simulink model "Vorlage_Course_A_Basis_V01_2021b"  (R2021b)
settings: Solver=FixedStepAuto  StartTime=0.0  StopTime=inf  FixedStep=1e-3  RelTol=1e-3
undefined symbols (not defined in the file): bin2dec
libraries: simulink x9, instrumentseriallib x3, eeGeneralControl x1

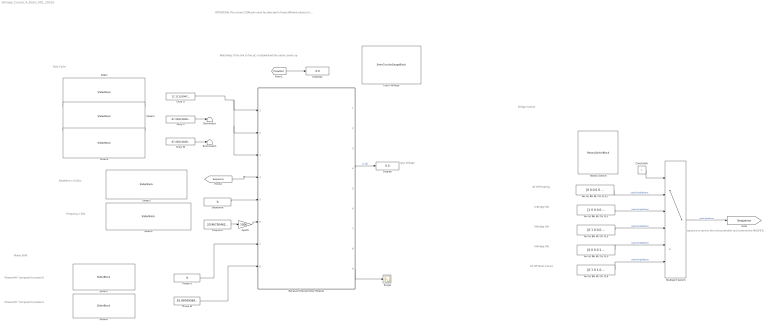
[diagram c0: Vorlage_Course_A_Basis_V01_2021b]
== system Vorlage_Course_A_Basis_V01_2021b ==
  note: Sequence is sent to the microcontroller and controls the MOSFETs
  note: Duty Cycle
  note: Phase Shift
  note: All Off Floating
  note: Watchdog: If the link to the µC is established the value counts up
  note: ATTENTION: The correct COM port must be selected in three different places in the receiver and transmitter module. (Available interfaces, see Windows Control Panel)
  note: Deadtime x 6,25ns
  note: Frequency / kHz
  note: Phaseshift °compared to phase U
  note: Phaseshift °compared to phase U
  note: U-Bridge ON
  note: V-Bridge ON
  note: V-Bridge ON
  note: All Off Short Circuit
  note: Bridge Control
  note: Input Voltage
  AH AL BH BL CH CL1 : Constant  Value=[1 0 0 0 0 0]  SampleTime=-1
  AH AL BH BL CH CL11 : Constant  Value=[0 0 0 0 0 0]  SampleTime=-1
  AH AL BH BL CH CL2 : Constant  Value=[0 1 0 0 0 0]  SampleTime=-1
  AH AL BH BL CH CL3 : Constant  Value=[0 0 0 0 1 0]  SampleTime=-1
  AH AL BH BL CH CL4 : Constant  Value=[0 1 0 1 0 1]
  Constant6 : Constant  OutDataTypeStr=uint8
  Deadtime : Constant  Value=0  OutDataTypeStr=uint16
  Display : Display
  Display1 : Display
  Duty U : Constant  Value=11.11110947376479
  Duty V : Constant  Value=67.2652182831598
  Duty W : Constant  Value=67.2652182831598
  Frequenz : Constant  Value=20.96730462519936  OutDataTypeStr=uint16
  Gain6 : Gain  Gain=1000
  Input Voltage : SemiCircularGaugeBlock  ScaleMax=25
  Multiport Switch : MultiPortSwitch  Inputs=5  DiagnosticForDefault=None
  Phase V : Constant  Value=0  OutDataTypeStr=uint16
  Phase W : Constant  Value=55.99769364620121  OutDataTypeStr=uint16
  Receiver/Transimmter Module : Subsystem
  Rotary Switch : RotarySwitchBlock
  Scope : Scope
  Slider : SliderBlock  TickInterval=20
  Slider1 : SliderBlock  TickInterval=20
  Slider2 : SliderBlock  TickInterval=20
  Slider3 : SliderBlock  ScaleMax=500  TickInterval=50
  Slider4 : SliderBlock  ScaleMin=1  ScaleMax=50  TickInterval=10
  Slider5 : SliderBlock  ScaleMax=180  TickInterval=20
  Slider6 : SliderBlock  ScaleMax=180  TickInterval=20
  Terminator : Terminator
  Terminator1 : Terminator
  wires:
  AH AL BH BL CH CL1/1 -> Multiport Switch/3  "switchingPattern"
  AH AL BH BL CH CL11/1 -> Multiport Switch/2  "switchingPattern"
  AH AL BH BL CH CL2/1 -> Multiport Switch/4  "switchingPattern"
  Multiport Switch/1 -> [Sequence]  "switchpattern"
  AH AL BH BL CH CL3/1 -> Multiport Switch/5  "switchingPattern"
  Constant6/1 -> Multiport Switch/1
  AH AL BH BL CH CL4/1 -> Multiport Switch/6  "switchingPattern"
  [Sequence] -> Receiver/Transimmter Module/4(Sequence UH UL VH VL WH WL)
  [Counter] -> Display1/1
  Duty U/1 -> Receiver/Transimmter Module/2(Duty V [%]), Receiver/Transimmter Module/3(Duty W [%]), Receiver/Transimmter Module/1(Duty U [%])
  Deadtime/1 -> Receiver/Transimmter Module/5(Deadtime [x6,25n])
  Frequenz/1 -> Gain6/1
  Gain6/1 -> Receiver/Transimmter Module/6(Frequency [Hz])
  Phase V/1 -> Receiver/Transimmter Module/7(Phase V - U [°])
  Phase W/1 -> Receiver/Transimmter Module/8(Phase W - U [°])
  Duty V/1 -> Terminator/1
  Duty W/1 -> Terminator1/1
  Receiver/Transimmter Module/4(U_ZK [V]) -> Display/1  "U_ZK"
  Receiver/Transimmter Module/9(Analog Sig) -> Scope/1

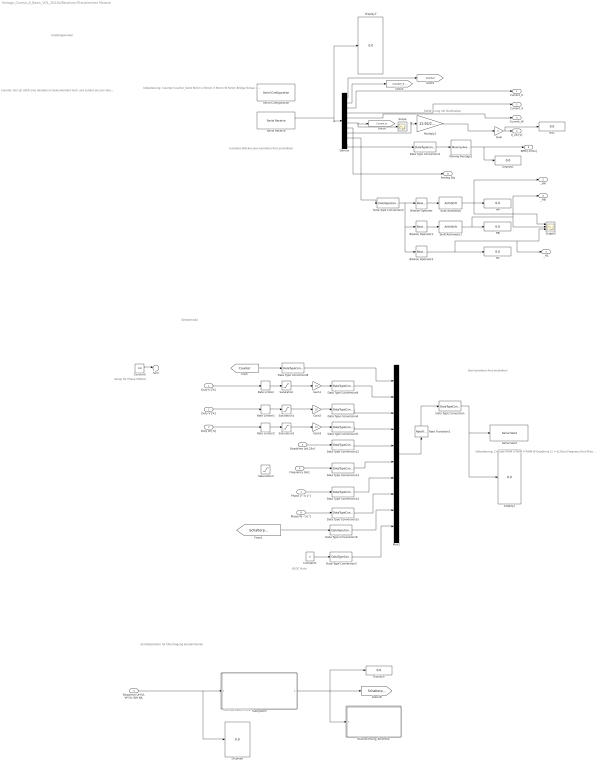
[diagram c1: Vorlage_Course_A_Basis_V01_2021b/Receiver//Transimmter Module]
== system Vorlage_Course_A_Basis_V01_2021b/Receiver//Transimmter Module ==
  note: BLDC Auto
  note: Setup für Phase-Shifted
  note: Counter: Der µC zählt eine Variable im Sekundentakt hoch und sendet sie zum Host Counter_Send: Der empfangene Wert wird wieder nach unten gesendet und sofort wieder empfangen Die Variable läuft ein mal im Kreis. Zählen beide Werte hoch ist alles in Ordnung. Zählt nur der Counter hoch bedeutet das, dass der Ursprungscounter nicht zurückgesendet wurde bzw. allgemein kein Daten von Simulink zum µC übertragen werden.
  note: Dekodierung: Counter Counter_Send Strom U Strom V Strom W Strom Bridge Torque U Zwischenkreis Hall Drehzahl
  note: Kalibrierung mit Oszilloskop
  note: Dekodierung: Counter PWM U PWM V PWM W Deadtime [1 = 6,25ns] Frequenz [Hz] Phase V PHase W Schaltsequenz BLDC Automatic
  note: Den korrekten Port einstellen!
  note: Sendemodul
  note: Empfangsmodul
  note: In beiden Blöcken den korrekten Port einstelllen!
  note: Schalterpattern für Übertragung komplrimieren
  note: Gibt das Pattern aus
  Duty U [%] : Inport
  Duty V [%] : Inport  Port=2
  Duty W [%] : Inport  Port=3
  Sequence UH UL VH VL WH WL : Inport  Port=4
  Deadtime [x6,25n] : Inport  Port=5
  Frequency [Hz] : Inport  Port=6
  Phase V - U [°] : Inport  Port=7
  Phase W - U [°] : Inport  Port=8
  Bitwise Operator : simulink/Logic and Bit Operations/Bitwise Operator  logicop=AND  UseBitMask=on  BitMask=bin2dec('00000100')  BitMaskRealWorld=Stored Integer
  Bitwise Operator1 : simulink/Logic and Bit Operations/Bitwise Operator  logicop=AND  UseBitMask=on  BitMask=bin2dec('00000010')  BitMaskRealWorld=Stored Integer
  Bitwise Operator2 : simulink/Logic and Bit Operations/Bitwise Operator  logicop=AND  UseBitMask=on  BitMask=bin2dec('00000001')  BitMaskRealWorld=Stored Integer
  Constant : Constant  Value=100
  Constant1 : Constant  Value=0
  Data Type Conversion{,3..5,8..9,12..16} (11 alike) : DataTypeConversion  OutDataTypeStr=uint16
  Data Type Conversion1 : DataTypeConversion  OutDataTypeStr=double
  Data Type Conversion2 : DataTypeConversion  OutDataTypeStr=uint8
  Demux : Demux  Outputs=10
  Display{1..2,5..7} (5 alike) : Display
  Gain : Gain
  Gain1 : Gain  Gain=10
  Gain2 : Gain  Gain=10
  Gain3 : Gain  Gain=10
  HA : Display
  HA1 : Display
  HB : Display
  HC : Display
  Moving Average1 : eeGeneralControl/Moving Average  VariantControl=Variant1  LabelModeActiveChoice=Discrete  f=2  x0=0  BufferSize=8192  Ts=-1
  Multiply1 : Gain  Gain=22.92/2366
  Mux2 : Mux  Inputs=10
  Rate Limiter : RateLimiter  RisingSlewLimit=200  FallingSlewLimit=-200
  Rate Limiter1 : RateLimiter  RisingSlewLimit=200  FallingSlewLimit=-200
  Rate Limiter2 : RateLimiter  RisingSlewLimit=200  FallingSlewLimit=-200
  Rate Transition1 : RateTransition  OutPortSampleTime=0.05
  Rückrechnung_Kontrolle : Subsystem
  Saturation : Saturate  UpperLimit=90  LowerLimit=0
  Saturation1 : Saturate  UpperLimit=90  LowerLimit=0
  Saturation2 : Saturate  UpperLimit=90  LowerLimit=0
  Saturation3 : Saturate  UpperLimit=100000  LowerLimit=1000
  Scope : Scope
  Scope3 : Scope  NumInputPorts=3
  Serial Configuration : instrumentseriallib/Serial Configuration  Priority=-200000  Port=COM22  ComPort=COM22  BaudRate=115000  DataBits=8  Parity=even  StopBits=1  ByteOrder=little-endian  FlowControl=none  Timeout=10  SimulateUsing=Interpreted execution  BlockInModel=on
  Serial Receive : instrumentseriallib/Serial Receive  Priority=1  Port=COM22  ComPort=COM22  DataType=uint16  SaveDataType=uint8  ToggleHeader=on  Header=['X']  ToggleTerminator=on  Terminator=Custom terminator  CustomTerminator=['Y']  ToggleDataSize=on  DataSize=[1 10]  EnableBlockingMode=off  ActionDataUnavailable=Output last received value  ActionWhenDataUnavailable=Output last received value  CustomValue=42  SampleTime=0.001  SimulateUsing=Interpreted execution  BlockInModel=on
  Serial Send : instrumentseriallib/Serial Send  Priority=1  Port=COM22  ComPort=COM22  Header=[]  Terminator=<none>  CustomTerminator=[]  EnableBlockingMode=off  SimulateUsing=Interpreted execution  BlockInModel=on
  Shift Arithmetic : ArithShift  BitShiftNumber=2  BitShiftDirection=Right
  Shift Arithmetic1 : ArithShift  BitShiftNumber=1  BitShiftDirection=Right
  Subsystem : Subsystem
  Sum : Sum  Inputs=|+-
  Current_U : Outport
  Current_V : Outport  Port=2
  Current_W : Outport  Port=3
  U_ZK [V] : Outport  Port=4
  _HA : Outport  Port=5
  _HB : Outport  Port=6
  _HC : Outport  Port=7
  " RPM [1/min]" : Outport  Port=8
  Analog Sig : Outport  Port=9
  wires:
  Demux/4 -> Current_V/1
  Data Type Conversion1/1 -> Moving Average1/1
  Serial Receive/1 -> Demux/1, Display7/1
  Demux/3 -> Current_U/1
  Moving Average1/1 -> " RPM [1/min]"/1, Display1/1
  Demux/5 -> Current_W/1
  Demux/6 -> Scope/1, [Current_In]
  Demux/2 -> [Counter_Send]
  Multiply1/1 -> Gain/1
  Demux/10 -> Data Type Conversion1/1
  Bitwise Operator1/1 -> Shift Arithmetic1/1
  Data Type Conversion2/1 -> Bitwise Operator2/1, Bitwise Operator1/1, Bitwise Operator/1
  Bitwise Operator/1 -> Shift Arithmetic/1
  Shift Arithmetic/1 -> _HA/1, Scope3/1, HA/1
  Shift Arithmetic1/1 -> _HB/1, Scope3/2, HB/1
  Bitwise Operator2/1 -> HC/1, _HC/1, Scope3/3
  Demux/8 -> Multiply1/1
  Demux/9 -> Data Type Conversion2/1
  Demux/1 -> [Counter]
  Data Type Conversion15/1 -> Mux2/8
  Data Type Conversion12/1 -> Mux2/5
  Data Type Conversion16/1 -> Mux2/9
  Data Type Conversion13/1 -> Mux2/6
  Data Type Conversion8/1 -> Mux2/1
  Data Type Conversion9/1 -> Mux2/2
  Rate Transition1/1 -> Data Type Conversion/1
  Mux2/1 -> Rate Transition1/1
  Gain1/1 -> Data Type Conversion9/1
  Duty U [%]/1 -> Rate Limiter/1
  Data Type Conversion/1 -> Display2/1, Serial Send/1
  Data Type Conversion14/1 -> Mux2/7
  Data Type Conversion3/1 -> Mux2/10
  [Counter] -> Data Type Conversion8/1
  Gain/1 -> HA1/1, U_ZK [V]/1
  Gain2/1 -> Data Type Conversion4/1
  Data Type Conversion4/1 -> Mux2/3
  Data Type Conversion5/1 -> Mux2/4
  Gain3/1 -> Data Type Conversion5/1
  Duty W [%]/1 -> Rate Limiter2/1
  Subsystem/1(Out1) -> Rückrechnung_Kontrolle/1(In1), [Schalterpattern], Display5/1
  Sequence UH UL VH VL WH WL/1 -> Display6/1, Subsystem/1(switchpattern)
  [Schalterpattern] -> Data Type Conversion16/1
  Rate Limiter/1 -> Saturation/1
  Rate Limiter1/1 -> Saturation1/1
  Rate Limiter2/1 -> Saturation2/1
  Constant/1 -> Sum/1
  Duty V [%]/1 -> Rate Limiter1/1
  Deadtime [x6,25n]/1 -> Data Type Conversion12/1
  Constant1/1 -> Data Type Conversion3/1
  Phase V - U [°]/1 -> Data Type Conversion14/1
  Phase W - U [°]/1 -> Data Type Conversion15/1
  Saturation/1 -> Gain1/1
  Saturation1/1 -> Gain2/1
  Saturation2/1 -> Gain3/1
  Frequency [Hz]/1 -> Data Type Conversion13/1
  Demux/7 -> Analog Sig/1

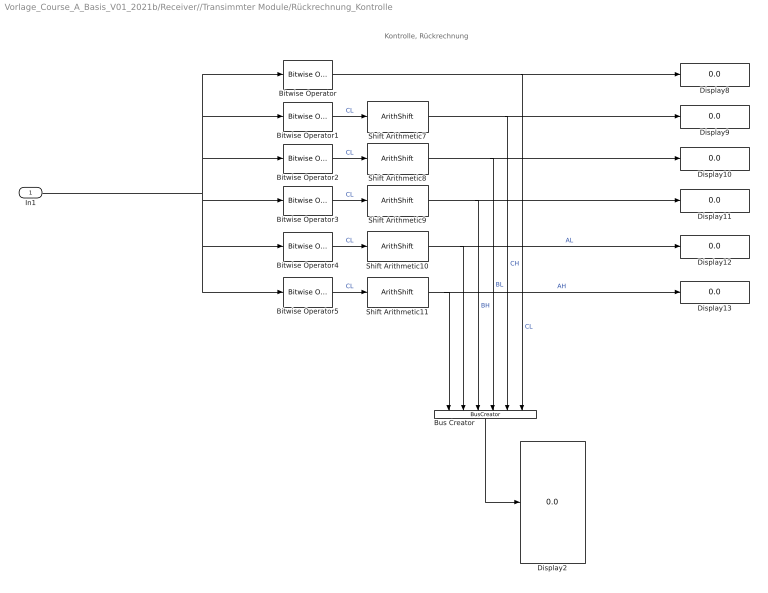
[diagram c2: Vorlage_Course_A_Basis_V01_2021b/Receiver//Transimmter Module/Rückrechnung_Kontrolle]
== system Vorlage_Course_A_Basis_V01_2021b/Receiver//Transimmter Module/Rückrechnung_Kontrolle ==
  note: Kontrolle, Rückrechnung
  In1 : Inport
  Bitwise Operator : simulink/Logic and Bit Operations/Bitwise Operator  logicop=AND  UseBitMask=on  BitMask=0x01  BitMaskRealWorld=Stored Integer
  Bitwise Operator1 : simulink/Logic and Bit Operations/Bitwise Operator  logicop=AND  UseBitMask=on  BitMask=0x02  BitMaskRealWorld=Stored Integer
  Bitwise Operator2 : simulink/Logic and Bit Operations/Bitwise Operator  logicop=AND  UseBitMask=on  BitMask=0x04  BitMaskRealWorld=Stored Integer
  Bitwise Operator3 : simulink/Logic and Bit Operations/Bitwise Operator  logicop=AND  UseBitMask=on  BitMask=0x08  BitMaskRealWorld=Stored Integer
  Bitwise Operator4 : simulink/Logic and Bit Operations/Bitwise Operator  logicop=AND  UseBitMask=on  BitMask=0x10  BitMaskRealWorld=Stored Integer
  Bitwise Operator5 : simulink/Logic and Bit Operations/Bitwise Operator  logicop=AND  UseBitMask=on  BitMask=0x20  BitMaskRealWorld=Stored Integer
  Bus Creator : BusCreator  Inputs=6
  Display{2,8..13} (7 alike) : Display
  Shift Arithmetic10 : ArithShift  BitShiftNumber=4  BitShiftDirection=Right
  Shift Arithmetic11 : ArithShift  BitShiftNumber=5  BitShiftDirection=Right
  Shift Arithmetic7 : ArithShift  BitShiftNumber=1  BitShiftDirection=Right
  Shift Arithmetic8 : ArithShift  BitShiftNumber=2  BitShiftDirection=Right
  Shift Arithmetic9 : ArithShift  BitShiftNumber=3  BitShiftDirection=Right
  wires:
  Shift Arithmetic8/1 -> Bus Creator/4, Display10/1  "BL"
  Shift Arithmetic9/1 -> Bus Creator/3, Display11/1  "BH"
  In1/1 -> Bitwise Operator/1, Bitwise Operator1/1, Bitwise Operator2/1, Bitwise Operator5/1, Bitwise Operator4/1, Bitwise Operator3/1
  Bitwise Operator2/1 -> Shift Arithmetic8/1  "CL"
  Shift Arithmetic7/1 -> Bus Creator/5, Display9/1  "CH"
  Shift Arithmetic10/1 -> Display12/1, Bus Creator/2  "AL"
  Bitwise Operator5/1 -> Shift Arithmetic11/1  "CL"
  Shift Arithmetic11/1 -> Display13/1, Bus Creator/1  "AH"
  Bitwise Operator/1 -> Bus Creator/6, Display8/1  "CL"
  Bus Creator/1 -> Display2/1
  Bitwise Operator1/1 -> Shift Arithmetic7/1  "CL"
  Bitwise Operator4/1 -> Shift Arithmetic10/1  "CL"
  Bitwise Operator3/1 -> Shift Arithmetic9/1  "CL"

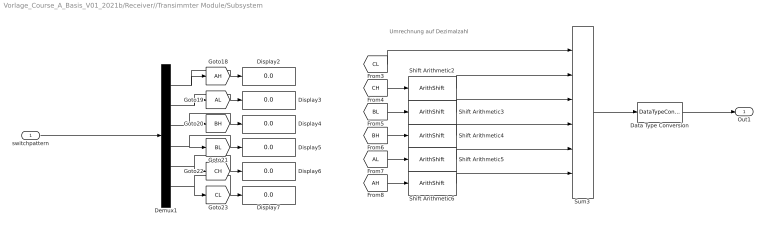
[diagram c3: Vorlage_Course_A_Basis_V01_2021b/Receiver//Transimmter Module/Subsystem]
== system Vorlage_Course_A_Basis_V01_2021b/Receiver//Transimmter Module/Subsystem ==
  note: Umrechnung auf Dezimalzahl
  switchpattern : Inport
  Data Type Conversion : DataTypeConversion  OutDataTypeStr=uint8
  Demux1 : Demux  Outputs=6
  Display{2..7} (6 alike) : Display
  Shift Arithmetic2 : ArithShift  BitShiftNumber=1  BitShiftDirection=Left
  Shift Arithmetic3 : ArithShift  BitShiftNumber=2  BitShiftDirection=Left
  Shift Arithmetic4 : ArithShift  BitShiftNumber=3  BitShiftDirection=Left
  Shift Arithmetic5 : ArithShift  BitShiftNumber=4  BitShiftDirection=Left
  Shift Arithmetic6 : ArithShift  BitShiftNumber=5  BitShiftDirection=Left
  Sum3 : Sum  Inputs=|++++++
  Out1 : Outport
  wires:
  [CL] -> Sum3/1
  Demux1/2 -> Display3/1, [AL]
  Demux1/4 -> [BL], Display5/1
  Demux1/5 -> Display6/1, [CH]
  Demux1/3 -> Display4/1, [BH]
  Shift Arithmetic4/1 -> Sum3/4
  Shift Arithmetic2/1 -> Sum3/2
  Demux1/1 -> [AH], Display2/1
  Data Type Conversion/1 -> Out1/1
  [AL] -> Shift Arithmetic5/1
  Demux1/6 -> Display7/1, [CL]
  [CH] -> Shift Arithmetic2/1
  Shift Arithmetic3/1 -> Sum3/3
  Shift Arithmetic6/1 -> Sum3/6
  [BH] -> Shift Arithmetic4/1
  [AH] -> Shift Arithmetic6/1
  Sum3/1 -> Data Type Conversion/1
  Shift Arithmetic5/1 -> Sum3/5
  [BL] -> Shift Arithmetic3/1
  switchpattern/1 -> Demux1/1
